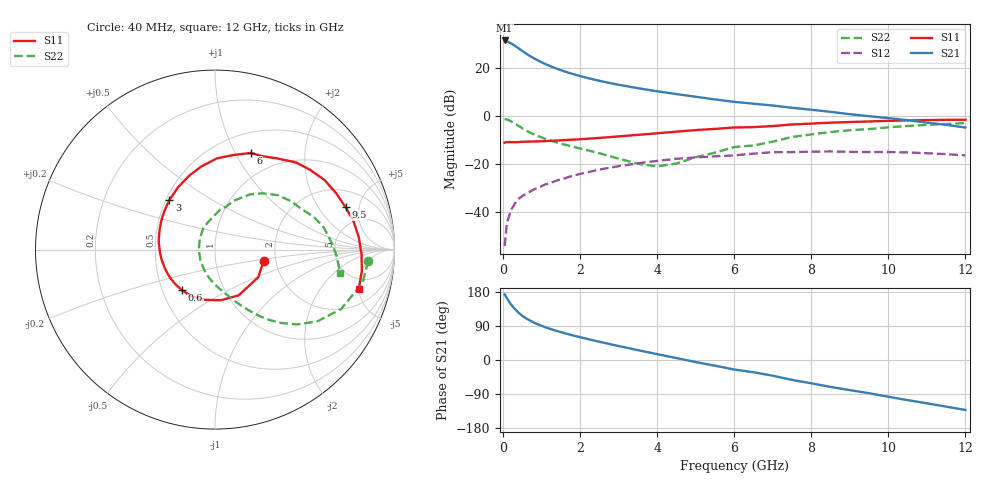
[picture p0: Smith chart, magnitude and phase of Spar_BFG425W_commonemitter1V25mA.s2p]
! Filename: 125bfg425.001
! BFG425W Field C1
! V1=8.814E-001V,V2=1.000E+000V, I1=3.896E-004A, I2=2.496E-002A
# GHz  S  MA  R 50
!  S11  S21  S12  S22
!Freq(GHz)  Mag  Ang  Mag  Ang  Mag  Ang  Mag  Ang
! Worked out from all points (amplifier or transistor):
!   44 points, 40 MHz to 12 GHz, reference 50 ohm
!   highest |S21| = 31.2 dB at 40 MHz (marker M1)
!   |S21| within 3 dB of that: start of sweep to 378.4 MHz
!   unconditionally stable (mu >= 1): start of sweep to 67.03 MHz; 984.7 MHz to end of sweep
!   at 700 MHz: K = 0.88, MSG = 28.1 dB, |S12| = -31.4 dB
!   at 2.4 GHz: K = 1.20, MAG = 16.1 dB, |S12| = -22.6 dB
!   at 12 GHz: K = 1.38, MAG = 2.1 dB, |S12| = -16.4 dB
!   S11 on the Smith chart (normalised r, x): 40 MHz: 1.72, -0.24; 600 MHz: 0.63, -0.31; 3 GHz: 0.52, +0.34; 6 GHz: 0.72, +1.16; 9.5 GHz: 3.19, +3.63; 12 GHz: 3.54, -5.02
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0.04  0.278 -13.1  36.44 173.2  0.002 75.1  0.855 -4.3
0.1  0.286 -32.7  35.28 163.1  0.006 79.8  0.843 -12.8
0.2  0.287 -62.7  31.78 147.3  0.011 72.7  0.777 -25.2
0.3  0.284 -83.5  28.57 135.2  0.015 68.3  0.697 -35.0
0.4  0.286 -102.0  25.08 125.0  0.019 64.4  0.62 -42.3
0.5  0.291 -117.3  22.03 116.5  0.022 62.4  0.552 -47.8
0.6  0.292 -128.9  19.46 109.7  0.024 61.0  0.497 -52.2
0.7  0.293 -138.3  17.33 103.9  0.027 59.8  0.451 -55.8
0.8  0.295 -146.6  15.57 98.7  0.03 59.2  0.413 -58.7
0.9  0.296 -153.6  14.12 94.2  0.032 58.5  0.383 -61.3
1.1  0.3 -165.2  11.82 86.4  0.038 57.1  0.334 -66.0
1.3  0.305 -174.5  10.13 79.6  0.043 55.5  0.296 -70.3
1.6  0.315 173.3  8.313 70.7  0.051 52.8  0.254 -76.4
2.2  0.336 154.0  6.06 55.3  0.068 46.1  0.193 -90.5
3  0.375 132.5  4.404 36.9  0.091 35.3  0.13 -116.8
4.5  0.47 99.1  2.827 5.1  0.129 12.0  0.103 145.9
6  0.574 69.7  1.949 -25.1  0.152 -13.0  0.226 82.4
6.5  0.584 63.0  1.787 -32.3  0.165 -17.3  0.244 76.0
8.5  0.723 32.4  1.211 -71.0  0.183 -53.3  0.463 41.0
9.5  0.765 18.0  0.985 -87.7  0.178 -69.1  0.533 24.9
10.5  0.804 4.9  0.813 -105.9  0.175 -86.6  0.619 11.4
12  0.831 -15.3  0.573 -131.8  0.152 -114.2  0.708 -10.4
